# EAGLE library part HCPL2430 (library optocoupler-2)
HEWLETT PACKARD OPTO COUPLER
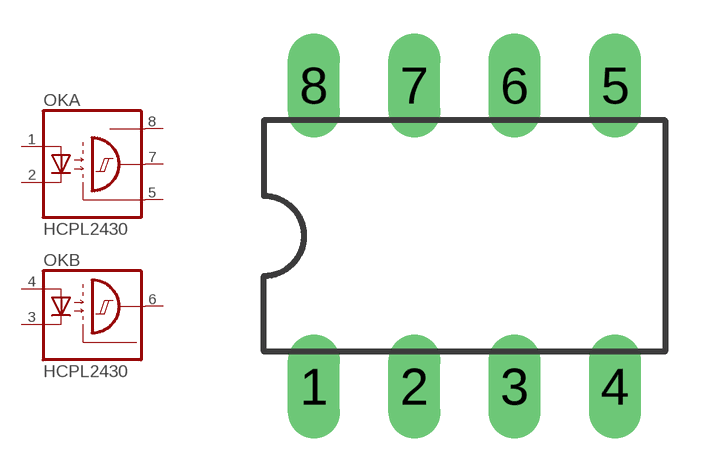
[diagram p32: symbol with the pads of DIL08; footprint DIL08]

Designator prefix OK; gates A=2231 B=2231A

## HCPL2430  [DIL08]
1  A:A  pas
2  A:C  pas
3  B:C  pas
4  B:A  pas
5  A:GND  pas
6  B:OUT  pas
7  A:OUT  pas
8  A:VCC  pas

## Footprint DIL08 (pad centres in mm)
Dual In Line Package
drill 0.813 long: 1 -3.81,-3.81; 2 -1.27,-3.81; 3 1.27,-3.81; 4 3.81,-3.81; 5 3.81,3.81; 6 1.27,3.81; 7 -1.27,3.81; 8 -3.81,3.81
